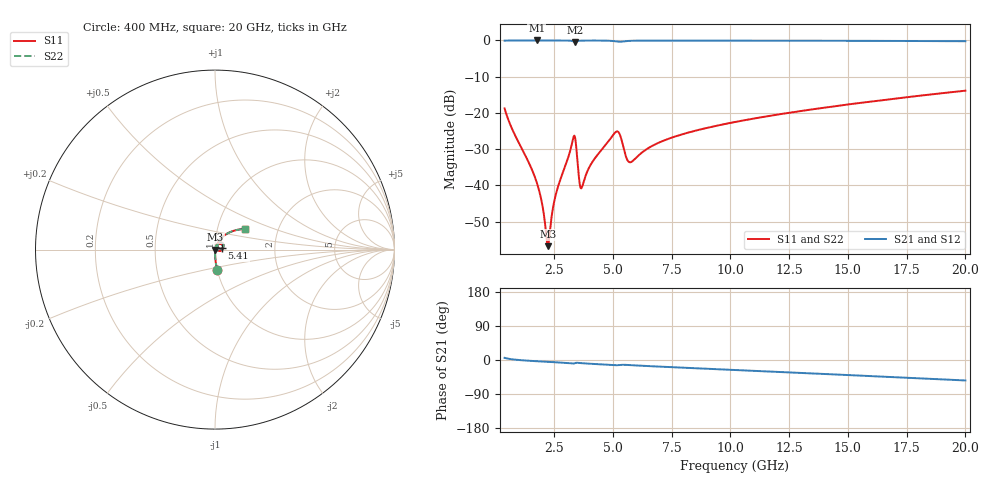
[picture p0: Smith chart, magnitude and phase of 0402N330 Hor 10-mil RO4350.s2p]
# MHz S  dB  R 50
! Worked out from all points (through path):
!   1961 points, 400 MHz to 20 GHz, reference 50 ohm
!   highest |S21| = -0.01 dB at 1.77 GHz (marker M1); lowest = -0.4 dB at 3.39 GHz (marker M2)
!   group delay of S21, straight-line fit = 7.72 ps
!   lowest |S11| = -56.8 dB at 2.24 GHz (marker M3), VSWR 1.00, Z = 50.1 - j0.0156 ohm
!   |S11| at or under -10 dB: start of sweep to end of sweep
!   |S22| runs from -56.8 to -13.9 dB; largest |S21 - S12| = 0
!   S11 on the Smith chart (normalised r, x): 400 MHz: 1.00, -0.23; 5.41 GHz: 1.08, +0.01; 20 GHz: 1.35, +0.33
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400  -18.77 -83.9  -0.06 5.7  -0.06 5.7  -18.77 -83.9
1770  -39.26 -86.8  -0.01 -3.3  -0.01 -3.3  -39.26 -86.8
1970  -44.24 -81.6  -0.01 -4.0  -0.01 -4.0  -44.24 -81.6
2180  -54.25 -47.8  -0.01 -4.7  -0.01 -4.7  -54.25 -47.8
2240  -56.76 -6.1  -0.01 -4.9  -0.01 -4.9  -56.76 -6.1
2300  -54.21 34.9  -0.01 -5.1  -0.01 -5.1  -54.21 34.9
2630  -41.27 71.5  -0.02 -6.2  -0.02 -6.2  -41.27 71.5
3300  -27.41 47.9  -0.21 -9.3  -0.21 -9.3  -27.41 47.9
3390  -26.60 11.7  -0.39 -8.3  -0.39 -8.3  -26.60 11.7
3580  -38.85 -5.6  -0.10 -7.9  -0.10 -7.9  -38.85 -5.6
3670  -40.74 30.3  -0.06 -8.4  -0.06 -8.4  -40.74 30.3
4120  -33.66 69.6  -0.04 -10.2  -0.04 -10.2  -33.66 69.6
5070  -25.63 50.4  -0.21 -13.8  -0.21 -13.8  -25.63 50.4
5250  -25.36 27.7  -0.37 -13.5  -0.37 -13.5  -25.36 27.7
5410  -28.33 10.3  -0.32 -12.7  -0.32 -12.7  -28.33 10.3
5590  -32.56 18.5  -0.18 -12.9  -0.18 -12.9  -32.56 18.5
5750  -33.61 38.1  -0.12 -13.5  -0.12 -13.5  -33.61 38.1
6940  -28.26 66.6  -0.04 -17.3  -0.04 -17.3  -28.26 66.6
10200  -22.51 61.1  -0.06 -26.4  -0.06 -26.4  -22.51 61.1
13470  -19.03 52.8  -0.09 -35.4  -0.09 -35.4  -19.03 52.8
16740  -16.26 44.0  -0.14 -44.6  -0.14 -44.6  -16.26 44.0
20000  -13.87 34.8  -0.23 -54.0  -0.23 -54.0  -13.87 34.8
